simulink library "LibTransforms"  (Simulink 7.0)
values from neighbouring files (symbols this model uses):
  a0 = 0.0    (= 0)    [quake.m]    (also in rampth.m = omega^3; rspect.m = 1; displA2T.m = positT2A(zeros(ntbl, 1), dof, rh, rb, rl, canon, atype); displEnvelope.m = varargin{1}{7})
  atype = []    [displA2T.m]    (also in displEnvelope.m = varargin{1}{6}; displJacobian.m = ones(nact, 1); displT2A.m; forceA2T.m)
  canon = [linDisplCanon linVelocCanon linAccelCanon linForceCanon  		 rotDisplCanon rotVelocCanon rotAccelCanon rotForceCanon]'    [initialize.m]    (also in accelEnvelope.m = varargin{1}{4}; displEnvelope.m = varargin{1}{5}; displPivotEnvelope.m = varargin{1}{6}; forceEnvelope.m = varargin{1}{6})
  dmax = ( (stroke2 + endLength2) * lengthCanon)'    [initialize.m]
  dof = [1 2]    [initialize.m]    (also in accelEnvelope.m = varargin{1}{1}; displEnvelope.m = varargin{1}{1}; displPivotEnvelope.m = varargin{1}{1}; forceEnvelope.m = varargin{1}{2})
  ea = dcm * ea    [initialize.m]    (also in accelEnvelope.m = varargin{1}{3})
  fmax = ( area1 * areaCanon * (supplyPress-returnPress) * pressCanon)'    [initialize.m]    (also in Tutorial.m = 50; forceEnvelope.m = varargin{1}{10}; forceJacobian.m = []; forceT2A.m = [])
  gee = geeCanon / linAccelCanon * 0    (= 0)    [initialize.m]    (also in accelA2T.m; accelEnvelope.m = varargin{1}{6}; accelT2A.m)
  linAccelCanon = 9810.0    (= 9810)    [initialize.m]    (also in accelJacobian.m = canon(3); accelP2Q.m = canon(3))
  linDisplCanon = 1    [initialize.m]    (also in displJacobian.m = canon(1); velocJacobian.m = canon(1))
  linVelocCanon = 1000.0    (= 1000)    [initialize.m]    (also in forceInvJacobian.m = canon(2); velocJacobian.m = canon(2); velocP2Q.m = canon(2))
  ra = dcm * ra    [initialize.m]    (also in accelEnvelope.m = varargin{1}{2})
  rb = dcm * rb    [initialize.m]    (also in displEnvelope.m = varargin{1}{3}; displPivotEnvelope.m = varargin{1}{3}; forceEnvelope.m = varargin{1}{4}; velocEnvelope.m = varargin{1}{4})
  rh = dcm * rh    [initialize.m]    (also in displEnvelope.m = varargin{1}{2}; displPivotEnvelope.m = varargin{1}{2}; forceEnvelope.m = varargin{1}{3}; velocEnvelope.m = varargin{1}{3})
  rl = dcm * rl    [initialize.m]    (also in displEnvelope.m = varargin{1}{4}; displPivotEnvelope.m = varargin{1}{4}; forceEnvelope.m = varargin{1}{5}; velocEnvelope.m = varargin{1}{5})
  rotAccelCanon = pi/180    (= 0.0174532925199)    [initialize.m]    (also in accelJacobian.m = canon(7); accelP2Q.m = canon(7); bodyAccel.m = canon(3); eulerAccel.m = canon(3))
  rotDisplCanon = pi/180    (= 0.0174532925199)    [initialize.m]    (also in accelA2T.m = canon(5); accelP2Q.m = canon(5); accelT2A.m = canon(5); bodyAccel.m = canon(1))
  rotForceCanon = 1000    [initialize.m]    (also in forceInvJacobian.m = canon(8); forceP2Q.m = canon(8))
  rotVelocCanon = pi/180    (= 0.0174532925199)    [initialize.m]    (also in accelJacobian.m = canon(6); accelP2Q.m = canon(6); bodyAccel.m = canon(2); eulerAccel.m = canon(2))
  rows = size(header, 1)    [player.m]    (also in quake.m; savebin.m; viewer.m; accelA2T.m = size(vrot, 1))
  rpq = rpq(:)    [accelP2Q.m]    (also in displP2Q.m; forceP2Q.m; velocP2Q.m)
undefined symbols (not defined in the file or in its folder): aijac, ajac, cols, Column, D, magnitude, matrix, vector
libraries: LibTransforms x99, aerospace x9, simulink x6
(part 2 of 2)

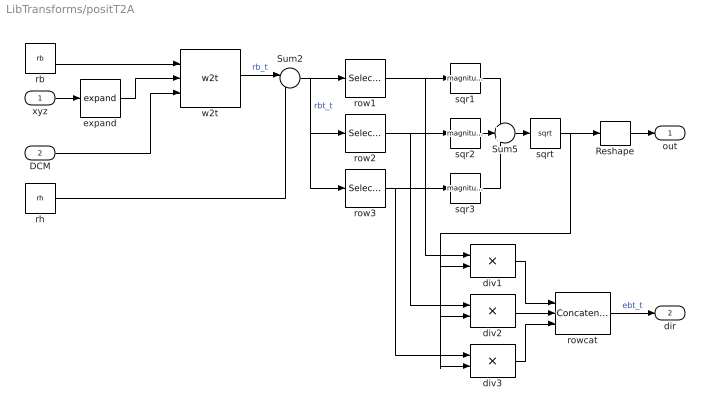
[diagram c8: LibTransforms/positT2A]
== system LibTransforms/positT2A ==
  xyz : Inport  OutDataType=sfix(16)  OutScaling=2^0
  DCM : Inport  Port=2  OutDataType=sfix(16)  OutScaling=2^0
  Reshape : Reshape
  Sum2 : Sum  Inputs=|-+  OutDataType=sfix(16)  OutScaling=2^0
  Sum5 : Sum  Inputs=+++  OutDataType=sfix(16)  OutScaling=2^0
  div1 : Product  Inputs=*/  OutDataType=sfix(16)  OutScaling=2^0
  div2 : Product  Inputs=*/  OutDataType=sfix(16)  OutScaling=2^0
  div3 : Product  Inputs=*/  OutDataType=sfix(16)  OutScaling=2^0
  expand : LibTransforms/expand  SystemSampleTime=-1  size=3  elements=dof(find(dof<=3))
  rb : Constant  Value=rb  OutDataType=sfix(16)  OutScaling=2^0
  rh : Constant  Value=rh  OutDataType=sfix(16)  OutScaling=2^0
  row1 : Selector  NumberOfDimensions=2  InputPortWidth=3  IndexOptions=Index vector (dialog),Select all  Indices=1,-1  OutputSizes=1
  row2 : Selector  NumberOfDimensions=2  InputPortWidth=3  IndexOptions=Index vector (dialog),Select all  Indices=2,-1  OutputSizes=1
  row3 : Selector  NumberOfDimensions=2  InputPortWidth=3  IndexOptions=Index vector (dialog),Select all  Indices=3,-1  OutputSizes=1
  rowcat : Concatenate  NumInputs=3  Mode=Multidimensional array
  sqr1 : Math  Operator=magnitude^2  OutDataType=sfix(16)  OutScaling=2^0
  sqr2 : Math  Operator=magnitude^2  OutDataType=sfix(16)  OutScaling=2^0
  sqr3 : Math  Operator=magnitude^2  OutDataType=sfix(16)  OutScaling=2^0
  sqrt : Math  Operator=sqrt  OutDataType=sfix(16)  OutScaling=2^0
  w2t : LibTransforms/w2t  SystemSampleTime=-1
  out : Outport  OutDataType=sfix(16)  OutScaling=2^0
  dir : Outport  Port=2  OutDataType=sfix(16)  OutScaling=2^0
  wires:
  expand/1 -> w2t/2
  xyz/1 -> expand/1
  rb/1 -> w2t/1
  rh/1 -> Sum2/2
  row2/1 -> sqr2/1, div2/1
  row1/1 -> sqr1/1, div1/1
  row3/1 -> sqr3/1, div3/1
  Sum5/1 -> sqrt/1
  sqrt/1 -> div1/2, div2/2, div3/2, Reshape/1
  w2t/1 -> Sum2/1  "rb_t"
  Sum2/1 -> row3/1, row2/1, row1/1  "rbt_t"
  sqr1/1 -> Sum5/1
  sqr2/1 -> Sum5/2
  sqr3/1 -> Sum5/3
  rowcat/1 -> dir/1  "ebt_t"
  div1/1 -> rowcat/1
  div2/1 -> rowcat/2
  div3/1 -> rowcat/3
  DCM/1 -> w2t/3
  Reshape/1 -> out/1

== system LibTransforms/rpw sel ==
  inp : Inport  OutDataType=sfix(16)  OutScaling=2^0
  Selector : Selector  IndexOptions=Index vector (dialog)  Indices=elements  OutputSizes=1
  out : Outport  OutDataType=sfix(16)  OutScaling=2^0
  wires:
  inp/1 -> Selector/1
  Selector/1 -> out/1

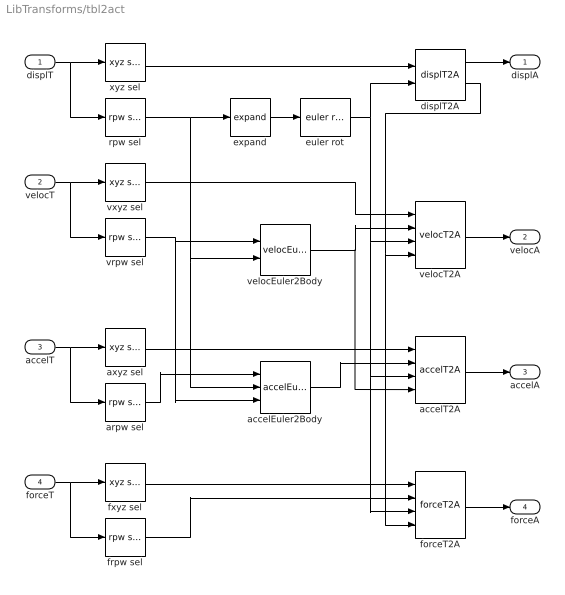
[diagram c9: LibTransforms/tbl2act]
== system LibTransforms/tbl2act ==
  displT : Inport  OutDataType=sfix(16)  OutScaling=2^0
  velocT : Inport  Port=2  OutDataType=sfix(16)  OutScaling=2^0
  accelT : Inport  Port=3  OutDataType=sfix(16)  OutScaling=2^0
  forceT : Inport  Port=4  OutDataType=sfix(16)  OutScaling=2^0
  accelEuler2Body : LibTransforms/accelEuler2Body  SystemSampleTime=-1  dof=dof
  accelT2A : LibTransforms/accelT2A  SystemSampleTime=-1  dof=dof  ra=ra  ea=ea  jac=ajac  gee=gee
  arpw sel : LibTransforms/rpw sel  SystemSampleTime=-1  dof=dof
  axyz sel : LibTransforms/xyz sel  SystemSampleTime=-1  dof=dof
  displT2A : LibTransforms/displT2A  SystemSampleTime=-1  dof=dof  rh=rh  rb=rb  a0=a0
  euler rot : LibTransforms/euler rot  SystemSampleTime=-1
  expand : LibTransforms/expand  SystemSampleTime=-1  size=3  elements=dof(find(dof>3))-3
  forceT2A : LibTransforms/forceT2A  SystemSampleTime=-1  dof=dof  rh=rh
  frpw sel : LibTransforms/rpw sel  SystemSampleTime=-1  dof=dof
  fxyz sel : LibTransforms/xyz sel  SystemSampleTime=-1  dof=dof
  rpw sel : LibTransforms/rpw sel  SystemSampleTime=-1  dof=dof
  velocEuler2Body : LibTransforms/velocEuler2Body  SystemSampleTime=-1  dof=dof
  velocT2A : LibTransforms/velocT2A  SystemSampleTime=-1  dof=dof  rh=rh
  vrpw sel : LibTransforms/rpw sel  SystemSampleTime=-1  dof=dof
  vxyz sel : LibTransforms/xyz sel  SystemSampleTime=-1  dof=dof
  xyz sel : LibTransforms/xyz sel  SystemSampleTime=-1  dof=dof
  displA : Outport  OutDataType=sfix(16)  OutScaling=2^0
  velocA : Outport  Port=2  OutDataType=sfix(16)  OutScaling=2^0
  accelA : Outport  Port=3  OutDataType=sfix(16)  OutScaling=2^0
  forceA : Outport  Port=4  OutDataType=sfix(16)  OutScaling=2^0
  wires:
  expand/1 -> euler rot/1
  xyz sel/1 -> displT2A/1
  displT/1 -> xyz sel/1, rpw sel/1
  rpw sel/1 -> expand/1, velocEuler2Body/2, accelEuler2Body/2
  euler rot/1 -> displT2A/2, accelT2A/3, forceT2A/3, velocT2A/3
  axyz sel/1 -> accelT2A/1
  accelT/1 -> arpw sel/1, axyz sel/1
  displT2A/2 -> forceT2A/4, velocT2A/4
  displT2A/1 -> displA/1
  forceT2A/1 -> forceA/1
  forceT/1 -> frpw sel/1, fxyz sel/1
  fxyz sel/1 -> forceT2A/1
  frpw sel/1 -> forceT2A/2
  velocEuler2Body/1 -> accelT2A/4, velocT2A/2
  accelEuler2Body/1 -> accelT2A/2
  arpw sel/1 -> accelEuler2Body/1
  accelT2A/1 -> accelA/1
  velocT/1 -> vrpw sel/1, vxyz sel/1
  vrpw sel/1 -> velocEuler2Body/1, accelEuler2Body/3
  velocT2A/1 -> velocA/1
  vxyz sel/1 -> velocT2A/1

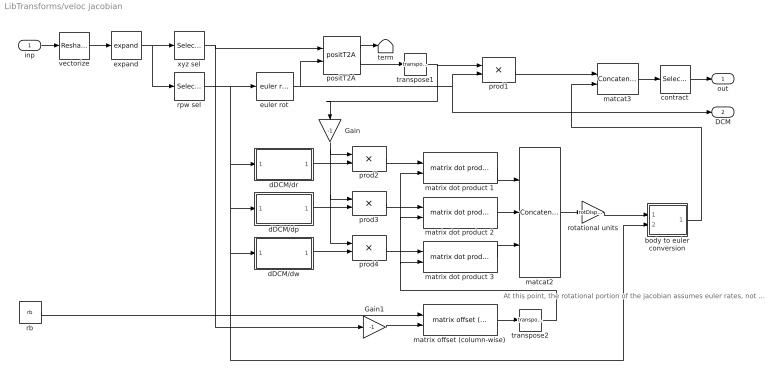
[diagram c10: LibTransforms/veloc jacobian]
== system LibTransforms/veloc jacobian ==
  note: At this point, the rotational portion of the jacobian assumes euler rates, not body rates. To convert it to use body rates, blend the body-to-euler transformation matrix into the rotational portion.
  inp : Inport  OutDataType=sfix(16)  OutScaling=2^0
  Gain : Gain  Orientation=down  Gain=-1  ParameterDataType=sfix(16)  ParameterScaling=2^0  OutDataType=sfix(16)  OutScaling=2^0
  Gain1 : Gain  Gain=-1  ParameterDataType=sfix(16)  ParameterScaling=2^0  OutDataType=sfix(16)  OutScaling=2^0
  body to euler conversion : Subsystem
  contract : Selector  NumberOfDimensions=2  InputPortWidth=3  IndexOptions=Select all,Index vector (dialog)  Indices=-1,dof  OutputSizes=1
  dDCM/dp : Subsystem
  dDCM/dr : Subsystem
  dDCM/dw : Subsystem
  euler rot : LibTransforms/euler rot  SystemSampleTime=-1
  expand : LibTransforms/expand  SystemSampleTime=-1  size=6  elements=dof
  matcat2 : Concatenate  NumInputs=3  Mode=Multidimensional array  ConcatenateDimension=2
  matcat3 : Concatenate  Mode=Multidimensional array  ConcatenateDimension=2
  matrix dot product 1 : LibTransforms/matrix dot product (row-wise)  SystemSampleTime=-1  rows=size(rh,2)
  matrix dot product 2 : LibTransforms/matrix dot product (row-wise)  SystemSampleTime=-1  rows=size(rh,2)
  matrix dot product 3 : LibTransforms/matrix dot product (row-wise)  SystemSampleTime=-1  rows=size(rh,2)
  matrix offset (column-wise) : LibTransforms/matrix offset (column-wise)  SystemSampleTime=-1  cols=size(rh,2)
  positT2A : LibTransforms/positT2A  SystemSampleTime=-1  dof=1:6  rh=rh  rb=rb
  prod{1..4} (4 alike) : Product  Multiplication=Matrix(*)  OutDataType=sfix(16)  OutScaling=2^0
  rb : Constant  Value=rb  OutDataType=sfix(16)  OutScaling=2^0
  rotational units : Gain  Gain=rotDisplCanon * (linDisplCanon/rotDisplCanon) * (rotVelocCanon/linVelocCanon)  ParameterDataType=sfix(16)  ParameterScaling=2^0  OutDataType=sfix(16)  OutScaling=2^0
  rpw sel : Selector  IndexOptions=Index vector (dialog)  Indices=[4 5 6]  OutputSizes=1
  term : Terminator
  transpose1 : Math  Operator=transpose  OutDataType=sfix(16)  OutScaling=2^0
  transpose2 : Math  Operator=transpose  OutDataType=sfix(16)  OutScaling=2^0
  vectorize : Reshape  OutputDimensionality=Column vector (2-D)  OutputDimensions=[3,3]
  xyz sel : Selector  IndexOptions=Index vector (dialog)  Indices=[1 2 3]  OutputSizes=1
  out : Outport  OutDataType=sfix(16)  OutScaling=2^0
  DCM : Outport  Port=2  OutDataType=sfix(16)  OutScaling=2^0
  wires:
  body to euler conversion/1(out) -> matcat3/2
  rb/1 -> matrix offset (column-wise)/1
  Gain1/1 -> matrix offset (column-wise)/2
  transpose2/1 -> matrix dot product 3/2, matrix dot product 2/2, matrix dot product 1/2
  rotational units/1 -> body to euler conversion/1(inp)
  matrix dot product 3/1 -> matcat2/3
  matrix dot product 2/1 -> matcat2/2
  matrix dot product 1/1 -> matcat2/1
  inp/1 -> vectorize/1
  rpw sel/1 -> body to euler conversion/2(rpw), dDCM/dw/1(rpw), dDCM/dp/1(rpw), dDCM/dr/1(rpw), euler rot/1
  euler rot/1 -> positT2A/2, prod1/2, DCM/1
  xyz sel/1 -> positT2A/1, Gain1/1
  positT2A/1 -> term/1
  dDCM/dr/1(dDCM/dr) -> prod2/2
  dDCM/dw/1(dDCM/dw) -> prod4/2
  dDCM/dp/1(dDCM/dp) -> prod3/2
  matrix offset (column-wise)/1 -> transpose2/1
  prod2/1 -> matrix dot product 1/1
  prod3/1 -> matrix dot product 2/1
  prod4/1 -> matrix dot product 3/1
  matcat2/1 -> rotational units/1
  prod1/1 -> matcat3/1
  matcat3/1 -> contract/1
  Gain/1 -> prod4/1, prod3/1, prod2/1
  positT2A/2 -> transpose1/1
  transpose1/1 -> prod1/1, Gain/1
  expand/1 -> rpw sel/1, xyz sel/1
  contract/1 -> out/1
  vectorize/1 -> expand/1

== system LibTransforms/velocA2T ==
  inp : Inport  OutDataType=sfix(16)  OutScaling=2^0
  dinp : Inport  Port=2  OutDataType=sfix(16)  OutScaling=2^0
  Terminator : Terminator
  matrix inverse : LibTransforms/matrix inverse  SystemSampleTime=-1  rows=size(rh, 2)  cols=length(dof)  wate=[]
  prod : Product  Multiplication=Matrix(*)  OutDataType=sfix(16)  OutScaling=2^0
  rpw sel : LibTransforms/rpw sel  SystemSampleTime=-1  dof=dof
  veloc jacobian : LibTransforms/veloc jacobian  SystemSampleTime=-1  dof=dof  rh=rh  rb=rb
  xyz sel : LibTransforms/xyz sel  SystemSampleTime=-1  dof=dof
  xyz : Outport  OutDataType=sfix(16)  OutScaling=2^0
  rpw : Outport  Port=2  OutDataType=sfix(16)  OutScaling=2^0
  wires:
  rpw sel/1 -> rpw/1
  prod/1 -> rpw sel/1, xyz sel/1
  matrix inverse/1 -> prod/1
  veloc jacobian/1 -> matrix inverse/1
  veloc jacobian/2 -> Terminator/1
  xyz sel/1 -> xyz/1
  dinp/1 -> veloc jacobian/1
  inp/1 -> prod/2

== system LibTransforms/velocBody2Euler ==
  inp : Inport  OutDataType=sfix(16)  OutScaling=2^0
  rpw : Inport  Port=2  OutDataType=sfix(16)  OutScaling=2^0
  contract : LibTransforms/contract  SystemSampleTime=-1  elements=[dof(find(dof>3))-3]
  euler rate : LibTransforms/euler rate  SystemSampleTime=-1
  expand 1 : LibTransforms/expand  SystemSampleTime=-1  size=3  elements=dof(find(dof>3))-3
  expand 2 : LibTransforms/expand  SystemSampleTime=-1  size=3  elements=dof(find(dof>3))-3
  out : Outport  OutDataType=sfix(16)  OutScaling=2^0
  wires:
  expand 2/1 -> euler rate/2
  expand 1/1 -> euler rate/1
  contract/1 -> out/1
  rpw/1 -> expand 2/1
  inp/1 -> expand 1/1
  euler rate/1 -> contract/1

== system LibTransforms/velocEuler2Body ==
  inp : Inport  OutDataType=sfix(16)  OutScaling=2^0
  rpw : Inport  Port=2  OutDataType=sfix(16)  OutScaling=2^0
  body rate : LibTransforms/body rate  SystemSampleTime=-1
  contract : LibTransforms/contract  SystemSampleTime=-1  elements=[dof(find(dof>3))-3]
  expand 1 : LibTransforms/expand  SystemSampleTime=-1  size=3  elements=dof(find(dof>3))-3
  expand 2 : LibTransforms/expand  SystemSampleTime=-1  size=3  elements=dof(find(dof>3))-3
  out : Outport  OutDataType=sfix(16)  OutScaling=2^0
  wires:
  body rate/1 -> contract/1
  inp/1 -> expand 1/1
  rpw/1 -> expand 2/1
  contract/1 -> out/1
  expand 1/1 -> body rate/1
  expand 2/1 -> body rate/2

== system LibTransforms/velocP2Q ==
  xyz : Inport  OutDataType=sfix(16)  OutScaling=2^0
  rpw : Inport  Port=2  OutDataType=sfix(16)  OutScaling=2^0
  DCM : Inport  Port=3  OutDataType=sfix(16)  OutScaling=2^0
  Sum : Sum  Inputs=++|  OutDataType=sfix(16)  OutScaling=2^0
  contract : LibTransforms/contract  SystemSampleTime=-1  elements=dof(find(dof<=3))
  crossprod : aerospace/Axes Transformations/3x3 cross product  SystemSampleTime=-1
  expand rpw : LibTransforms/expand  SystemSampleTime=-1  size=3  elements=dof(find(dof>3)) - 3
  expand xyz : LibTransforms/expand  SystemSampleTime=-1  size=3  elements=dof(find(dof<=3))
  linVelocUnits : Gain  Gain=1/linVelocCanon  ParameterDataType=sfix(16)  ParameterScaling=2^0  OutDataType=sfix(16)  OutScaling=2^0
  origin offset : Constant  Value=ofst  OutDataType=sfix(16)  OutScaling=2^0
  prod : Product  Multiplication=Matrix(*)  OutDataType=sfix(16)  OutScaling=2^0
  rotVelocCanon : Gain  Gain=rotVelocCanon  ParameterDataType=sfix(16)  ParameterScaling=2^0  OutDataType=sfix(16)  OutScaling=2^0
  t2w : Math  Operator=transpose  OutDataType=sfix(16)  OutScaling=2^0
  out : Outport  OutDataType=sfix(16)  OutScaling=2^0
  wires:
  xyz/1 -> expand xyz/1
  linVelocUnits/1 -> Sum/2
  origin offset/1 -> crossprod/2
  expand rpw/1 -> crossprod/1
  rotVelocCanon/1 -> expand rpw/1
  rpw/1 -> rotVelocCanon/1
  DCM/1 -> t2w/1
  Sum/1 -> contract/1
  crossprod/1 -> prod/2
  t2w/1 -> prod/1
  expand xyz/1 -> Sum/1
  prod/1 -> linVelocUnits/1
  contract/1 -> out/1

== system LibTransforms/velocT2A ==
  xyz : Inport  OutDataType=sfix(16)  OutScaling=2^0
  rpw : Inport  Port=2  OutDataType=sfix(16)  OutScaling=2^0
  DCM : Inport  Port=3  OutDataType=sfix(16)  OutScaling=2^0
  dir : Inport  Port=4  OutDataType=sfix(16)  OutScaling=2^0
  subsystem : Subsystem
  out : Outport  OutDataType=sfix(16)  OutScaling=2^0
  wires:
  subsystem/1(out) -> out/1
  dir/1 -> subsystem/4(dir)
  xyz/1 -> subsystem/1(xyz)
  rpw/1 -> subsystem/2(rpw)
  DCM/1 -> subsystem/3(DCM)

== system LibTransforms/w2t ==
  inp : Inport  OutDataType=sfix(16)  OutScaling=2^0
  xyz : Inport  Port=2  OutDataType=sfix(16)  OutScaling=2^0
  DCM : Inport  Port=3  OutDataType=sfix(16)  OutScaling=2^0
  Demux : Demux  Outputs=3
  Sum5 : Sum  Inputs=-+|  OutDataType=sfix(16)  OutScaling=2^0
  Sum6 : Sum  Inputs=-+|  OutDataType=sfix(16)  OutScaling=2^0
  Sum7 : Sum  Inputs=-+|  OutDataType=sfix(16)  OutScaling=2^0
  prod : Product  Multiplication=Matrix(*)  OutDataType=sfix(16)  OutScaling=2^0
  row1A : Selector  NumberOfDimensions=2  InputPortWidth=3  IndexOptions=Index vector (dialog),Select all  Indices=1,-1  OutputSizes=1
  row2A : Selector  NumberOfDimensions=2  InputPortWidth=3  IndexOptions=Index vector (dialog),Select all  Indices=2,-1  OutputSizes=1
  row3A : Selector  NumberOfDimensions=2  InputPortWidth=3  IndexOptions=Index vector (dialog),Select all  Indices=3,-1  OutputSizes=1
  rowcat : Concatenate  NumInputs=3  Mode=Multidimensional array
  out : Outport  OutDataType=sfix(16)  OutScaling=2^0
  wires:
  Sum7/1 -> rowcat/3
  Sum5/1 -> rowcat/1
  Sum6/1 -> rowcat/2
  Demux/3 -> Sum7/1
  Demux/2 -> Sum6/1
  row3A/1 -> Sum7/2
  row2A/1 -> Sum6/2
  Demux/1 -> Sum5/1
  row1A/1 -> Sum5/2
  xyz/1 -> Demux/1
  inp/1 -> row1A/1, row2A/1, row3A/1
  rowcat/1 -> prod/2
  prod/1 -> out/1
  DCM/1 -> prod/1

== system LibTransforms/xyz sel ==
  inp : Inport  OutDataType=sfix(16)  OutScaling=2^0
  Selector : Selector  IndexOptions=Index vector (dialog)  Indices=elements  OutputSizes=1
  out : Outport  OutDataType=sfix(16)  OutScaling=2^0
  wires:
  Selector/1 -> out/1
  inp/1 -> Selector/1

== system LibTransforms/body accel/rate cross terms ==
  inp : Inport  OutDataType=sfix(16)  OutScaling=2^0
  13 : Fcn  Expr=-cos(u[2])*u[5]*u[6]
  23 : Fcn  Expr=-sin(u[1])*u[4]*u[5] + cos(u[1])*cos(u[2])*u[4]*u[6] - sin(u[1])*sin(u[2])*u[5]*u[6]
  33 : Fcn  Expr=-cos(u[1])*u[4]*u[5] - sin(u[1])*cos(u[2])*u[4]*u[6] - cos(u[1])*sin(u[2])*u[5]*u[6]
  Mux : Mux  Inputs=3
  out : Outport  OutDataType=sfix(16)  OutScaling=2^0
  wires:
  Mux/1 -> out/1
  33/1 -> Mux/3
  23/1 -> Mux/2
  13/1 -> Mux/1
  inp/1 -> 33/1, 23/1, 13/1

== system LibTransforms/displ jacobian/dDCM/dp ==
  rpw : Inport  OutDataType=sfix(16)  OutScaling=2^0
  11 : Fcn  Expr=-sin(u[2])*cos(u[3])
  12 : Fcn  Expr=-sin(u[2])*sin(u[3])
  13 : Fcn  Expr=-cos(u[2])
  21 : Fcn  Expr=sin(u[1])*cos(u[2])*cos(u[3])
  22 : Fcn  Expr=sin(u[1])*cos(u[2])*sin(u[3])
  23 : Fcn  Expr=-sin(u[1])*sin(u[2])
  31 : Fcn  Expr=cos(u[1])*cos(u[2])*cos(u[3])
  32 : Fcn  Expr=cos(u[1])*cos(u[2])*sin(u[3])
  33 : Fcn  Expr=-cos(u[1])*sin(u[2])
  9x1->3x3 : simulink/Math Operations/Reshape  OutputDimensionality=Customize  OutputDimensions=[3,3]
  Mux2 : Mux  Orientation=down  Inputs=9
  rotDisplCanon : Gain  Gain=rotDisplCanon  ParameterDataType=sfix(16)  ParameterScaling=2^0  OutDataType=sfix(16)  OutScaling=2^0
  dDCM/dp : Outport  OutDataType=sfix(16)  OutScaling=2^0
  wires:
  rotDisplCanon/1 -> 31/1, 21/1, 11/1, 32/1, 22/1, 12/1, 33/1, 23/1, 13/1
  9x1->3x3/1 -> dDCM/dp/1
  11/1 -> Mux2/1
  21/1 -> Mux2/2
  31/1 -> Mux2/3
  rpw/1 -> rotDisplCanon/1
  12/1 -> Mux2/4
  22/1 -> Mux2/5
  32/1 -> Mux2/6
  Mux2/1 -> 9x1->3x3/1
  13/1 -> Mux2/7
  23/1 -> Mux2/8
  33/1 -> Mux2/9

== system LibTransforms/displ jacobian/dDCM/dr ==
  rpw : Inport  OutDataType=sfix(16)  OutScaling=2^0
  11 : Fcn  Expr=0
  12 : Fcn  Expr=0
  13 : Fcn  Expr=0
  21 : Fcn  Expr=cos(u[1])*sin(u[2])*cos(u[3])+sin(u[1])*sin(u[3])
  22 : Fcn  Expr=cos(u[1])*sin(u[2])*sin(u[3])-sin(u[1])*cos(u[3])
  23 : Fcn  Expr=cos(u[1])*cos(u[2])
  31 : Fcn  Expr=-sin(u[1])*sin(u[2])*cos(u[3])+cos(u[1])*sin(u[3])
  32 : Fcn  Expr=-sin(u[1])*sin(u[2])*sin(u[3])-cos(u[1])*cos(u[3])
  33 : Fcn  Expr=-sin(u[1])*cos(u[2])
  9x1->3x3 : simulink/Math Operations/Reshape  OutputDimensionality=Customize  OutputDimensions=[3,3]
  Mux2 : Mux  Orientation=down  Inputs=9
  rotDisplCanon : Gain  Gain=rotDisplCanon  ParameterDataType=sfix(16)  ParameterScaling=2^0  OutDataType=sfix(16)  OutScaling=2^0
  dDCM/dr : Outport  OutDataType=sfix(16)  OutScaling=2^0
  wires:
  rotDisplCanon/1 -> 31/1, 21/1, 11/1, 32/1, 22/1, 12/1, 33/1, 23/1, 13/1
  9x1->3x3/1 -> dDCM/dr/1
  11/1 -> Mux2/1
  21/1 -> Mux2/2
  31/1 -> Mux2/3
  rpw/1 -> rotDisplCanon/1
  12/1 -> Mux2/4
  22/1 -> Mux2/5
  32/1 -> Mux2/6
  Mux2/1 -> 9x1->3x3/1
  13/1 -> Mux2/7
  23/1 -> Mux2/8
  33/1 -> Mux2/9

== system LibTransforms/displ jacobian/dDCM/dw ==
  rpw : Inport  OutDataType=sfix(16)  OutScaling=2^0
  11 : Fcn  Expr=-cos(u[2])*sin(u[3])
  12 : Fcn  Expr=cos(u[2])*cos(u[3])
  13 : Fcn  Expr=0
  21 : Fcn  Expr=-sin(u[1])*sin(u[2])*sin(u[3])-cos(u[1])*cos(u[3])
  22 : Fcn  Expr=sin(u[1])*sin(u[2])*cos(u[3])-cos(u[1])*sin(u[3])
  23 : Fcn  Expr=0
  31 : Fcn  Expr=-cos(u[1])*sin(u[2])*sin(u[3])+sin(u[1])*cos(u[3])
  32 : Fcn  Expr=cos(u[1])*sin(u[2])*cos(u[3])+sin(u[1])*sin(u[3])
  33 : Fcn  Expr=0
  9x1->3x3 : simulink/Math Operations/Reshape  OutputDimensionality=Customize  OutputDimensions=[3,3]
  Mux2 : Mux  Orientation=down  Inputs=9
  rotDisplCanon : Gain  Gain=rotDisplCanon  ParameterDataType=sfix(16)  ParameterScaling=2^0  OutDataType=sfix(16)  OutScaling=2^0
  dDCM/dw : Outport  OutDataType=sfix(16)  OutScaling=2^0
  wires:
  rotDisplCanon/1 -> 31/1, 21/1, 11/1, 32/1, 22/1, 12/1, 33/1, 23/1, 13/1
  9x1->3x3/1 -> dDCM/dw/1
  11/1 -> Mux2/1
  21/1 -> Mux2/2
  31/1 -> Mux2/3
  rpw/1 -> rotDisplCanon/1
  12/1 -> Mux2/4
  22/1 -> Mux2/5
  32/1 -> Mux2/6
  Mux2/1 -> 9x1->3x3/1
  13/1 -> Mux2/7
  23/1 -> Mux2/8
  33/1 -> Mux2/9

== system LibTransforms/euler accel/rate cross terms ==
  inp : Inport  OutDataType=sfix(16)  OutScaling=2^0
  13 : Fcn  Expr=tan(u[2])*u[4]*u[5] + (1/cos(u[2]))*u[5]*u[6]
  23 : Fcn  Expr=-cos(u[2])*u[4]*u[6]
  33 : Fcn  Expr=tan(u[2])*u[5]*u[6] + (1/cos(u[2]))*u[4]*u[5]
  Mux : Mux  Inputs=3
  out : Outport  OutDataType=sfix(16)  OutScaling=2^0
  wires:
  inp/1 -> 13/1, 23/1, 33/1
  13/1 -> Mux/1
  23/1 -> Mux/2
  33/1 -> Mux/3
  Mux/1 -> out/1

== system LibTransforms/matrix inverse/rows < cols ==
  inp : Inport  OutDataType=sfix(16)  OutScaling=2^0
  Action Port : ActionPort
  Product : Product  Multiplication=Matrix(*)  OutDataType=sfix(16)  OutScaling=2^0
  Product1 : Product  Multiplication=Matrix(*)  OutDataType=sfix(16)  OutScaling=2^0
  Product2 : Product  Multiplication=Matrix(*)  OutDataType=sfix(16)  OutScaling=2^0
  matrix inverse : Product  Inputs=/  Multiplication=Matrix(*)  OutDataType=sfix(16)  OutScaling=2^-10
  transpose1 : Math  Operator=transpose  OutDataType=sfix(16)  OutScaling=2^0
  weight : Constant  Value=w1  OutDataType=sfix(16)  OutScaling=2^0
  out : Outport  OutDataType=sfix(16)  OutScaling=2^0
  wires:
  matrix inverse/1 -> Product1/2
  Product2/1 -> Product1/1, Product/2
  weight/1 -> Product2/1
  transpose1/1 -> Product2/2
  Product/1 -> matrix inverse/1
  inp/1 -> Product/1, transpose1/1
  Product1/1 -> out/1

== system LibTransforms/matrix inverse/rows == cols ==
  inp : Inport  OutDataType=sfix(16)  OutScaling=2^0
  Action Port : ActionPort
  Product : Product  Multiplication=Matrix(*)  OutDataType=sfix(16)  OutScaling=2^0
  Product1 : Product  Multiplication=Matrix(*)  OutDataType=sfix(16)  OutScaling=2^0
  matrix inverse : Product  Inputs=/  Multiplication=Matrix(*)  OutDataType=sfix(16)  OutScaling=2^-10
  transpose1 : Math  Operator=transpose  OutDataType=sfix(16)  OutScaling=2^0
  out : Outport  OutDataType=sfix(16)  OutScaling=2^0
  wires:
  Product/1 -> matrix inverse/1
  inp/1 -> Product/2, transpose1/1
  matrix inverse/1 -> Product1/1
  transpose1/1 -> Product1/2, Product/1
  Product1/1 -> out/1

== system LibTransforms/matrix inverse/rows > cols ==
  inp : Inport  OutDataType=sfix(16)  OutScaling=2^0
  Action Port : ActionPort
  Product : Product  Multiplication=Matrix(*)  OutDataType=sfix(16)  OutScaling=2^0
  Product1 : Product  Multiplication=Matrix(*)  OutDataType=sfix(16)  OutScaling=2^0
  Product2 : Product  Multiplication=Matrix(*)  OutDataType=sfix(16)  OutScaling=2^0
  matrix inverse : Product  Inputs=/  Multiplication=Matrix(*)  OutDataType=sfix(16)  OutScaling=2^-10
  transpose1 : Math  Operator=transpose  OutDataType=sfix(16)  OutScaling=2^0
  weight : Constant  Value=w2  OutDataType=sfix(16)  OutScaling=2^0
  out : Outport  OutDataType=sfix(16)  OutScaling=2^0
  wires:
  matrix inverse/1 -> Product1/1
  Product2/1 -> Product1/2, Product/1
  weight/1 -> Product2/2
  transpose1/1 -> Product2/1
  inp/1 -> Product/2, transpose1/1
  Product/1 -> matrix inverse/1
  Product1/1 -> out/1

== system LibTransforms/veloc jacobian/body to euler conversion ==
  inp : Inport
  rpw : Inport  Port=2
  body2euler : LibTransforms/body2euler  SystemSampleTime=-1
  prod : Product  Multiplication=Matrix(*)  OutDataType=sfix(16)  OutScaling=2^0
  rotDisplCanon : Gain  Gain=rotDisplCanon  ParameterDataType=sfix(16)  ParameterScaling=2^0  OutDataType=sfix(16)  OutScaling=2^0
  out : Outport
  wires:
  rpw/1 -> rotDisplCanon/1
  prod/1 -> out/1
  inp/1 -> prod/1
  body2euler/1 -> prod/2
  rotDisplCanon/1 -> body2euler/1

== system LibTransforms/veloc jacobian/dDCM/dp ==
  rpw : Inport  OutDataType=sfix(16)  OutScaling=2^0
  11 : Fcn  Expr=-sin(u[2])*cos(u[3])
  12 : Fcn  Expr=-sin(u[2])*sin(u[3])
  13 : Fcn  Expr=-cos(u[2])
  21 : Fcn  Expr=sin(u[1])*cos(u[2])*cos(u[3])
  22 : Fcn  Expr=sin(u[1])*cos(u[2])*sin(u[3])
  23 : Fcn  Expr=-sin(u[1])*sin(u[2])
  31 : Fcn  Expr=cos(u[1])*cos(u[2])*cos(u[3])
  32 : Fcn  Expr=cos(u[1])*cos(u[2])*sin(u[3])
  33 : Fcn  Expr=-cos(u[1])*sin(u[2])
  9x1->3x3 : Reshape  OutputDimensionality=Customize  OutputDimensions=[3,3]
  Mux2 : Mux  Orientation=down  Inputs=9
  rotDisplCanon : Gain  Gain=rotDisplCanon  ParameterDataType=sfix(16)  ParameterScaling=2^0  OutDataType=sfix(16)  OutScaling=2^0
  dDCM/dp : Outport  OutDataType=sfix(16)  OutScaling=2^0
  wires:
  33/1 -> Mux2/9
  23/1 -> Mux2/8
  13/1 -> Mux2/7
  Mux2/1 -> 9x1->3x3/1
  32/1 -> Mux2/6
  22/1 -> Mux2/5
  12/1 -> Mux2/4
  rpw/1 -> rotDisplCanon/1
  31/1 -> Mux2/3
  21/1 -> Mux2/2
  11/1 -> Mux2/1
  9x1->3x3/1 -> dDCM/dp/1
  rotDisplCanon/1 -> 13/1, 23/1, 33/1, 12/1, 22/1, 32/1, 11/1, 21/1, 31/1

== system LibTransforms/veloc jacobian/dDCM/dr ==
  rpw : Inport  OutDataType=sfix(16)  OutScaling=2^0
  11 : Fcn  Expr=0
  12 : Fcn  Expr=0
  13 : Fcn  Expr=0
  21 : Fcn  Expr=cos(u[1])*sin(u[2])*cos(u[3])+sin(u[1])*sin(u[3])
  22 : Fcn  Expr=cos(u[1])*sin(u[2])*sin(u[3])-sin(u[1])*cos(u[3])
  23 : Fcn  Expr=cos(u[1])*cos(u[2])
  31 : Fcn  Expr=-sin(u[1])*sin(u[2])*cos(u[3])+cos(u[1])*sin(u[3])
  32 : Fcn  Expr=-sin(u[1])*sin(u[2])*sin(u[3])-cos(u[1])*cos(u[3])
  33 : Fcn  Expr=-sin(u[1])*cos(u[2])
  9x1->3x3 : Reshape  OutputDimensionality=Customize  OutputDimensions=[3,3]
  Mux2 : Mux  Orientation=down  Inputs=9
  rotDisplCanon : Gain  Gain=rotDisplCanon  ParameterDataType=sfix(16)  ParameterScaling=2^0  OutDataType=sfix(16)  OutScaling=2^0
  dDCM/dr : Outport  OutDataType=sfix(16)  OutScaling=2^0
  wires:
  33/1 -> Mux2/9
  23/1 -> Mux2/8
  13/1 -> Mux2/7
  Mux2/1 -> 9x1->3x3/1
  32/1 -> Mux2/6
  22/1 -> Mux2/5
  12/1 -> Mux2/4
  rpw/1 -> rotDisplCanon/1
  31/1 -> Mux2/3
  21/1 -> Mux2/2
  11/1 -> Mux2/1
  9x1->3x3/1 -> dDCM/dr/1
  rotDisplCanon/1 -> 13/1, 23/1, 33/1, 12/1, 22/1, 32/1, 11/1, 21/1, 31/1

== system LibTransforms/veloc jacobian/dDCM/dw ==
  rpw : Inport  OutDataType=sfix(16)  OutScaling=2^0
  11 : Fcn  Expr=-cos(u[2])*sin(u[3])
  12 : Fcn  Expr=cos(u[2])*cos(u[3])
  13 : Fcn  Expr=0
  21 : Fcn  Expr=-sin(u[1])*sin(u[2])*sin(u[3])-cos(u[1])*cos(u[3])
  22 : Fcn  Expr=sin(u[1])*sin(u[2])*cos(u[3])-cos(u[1])*sin(u[3])
  23 : Fcn  Expr=0
  31 : Fcn  Expr=-cos(u[1])*sin(u[2])*sin(u[3])+sin(u[1])*cos(u[3])
  32 : Fcn  Expr=cos(u[1])*sin(u[2])*cos(u[3])+sin(u[1])*sin(u[3])
  33 : Fcn  Expr=0
  9x1->3x3 : Reshape  OutputDimensionality=Customize  OutputDimensions=[3,3]
  Mux2 : Mux  Orientation=down  Inputs=9
  rotDisplCanon : Gain  Gain=rotDisplCanon  ParameterDataType=sfix(16)  ParameterScaling=2^0  OutDataType=sfix(16)  OutScaling=2^0
  dDCM/dw : Outport  OutDataType=sfix(16)  OutScaling=2^0
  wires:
  33/1 -> Mux2/9
  23/1 -> Mux2/8
  13/1 -> Mux2/7
  Mux2/1 -> 9x1->3x3/1
  32/1 -> Mux2/6
  22/1 -> Mux2/5
  12/1 -> Mux2/4
  rpw/1 -> rotDisplCanon/1
  31/1 -> Mux2/3
  21/1 -> Mux2/2
  11/1 -> Mux2/1
  9x1->3x3/1 -> dDCM/dw/1
  rotDisplCanon/1 -> 13/1, 23/1, 33/1, 12/1, 22/1, 32/1, 11/1, 21/1, 31/1

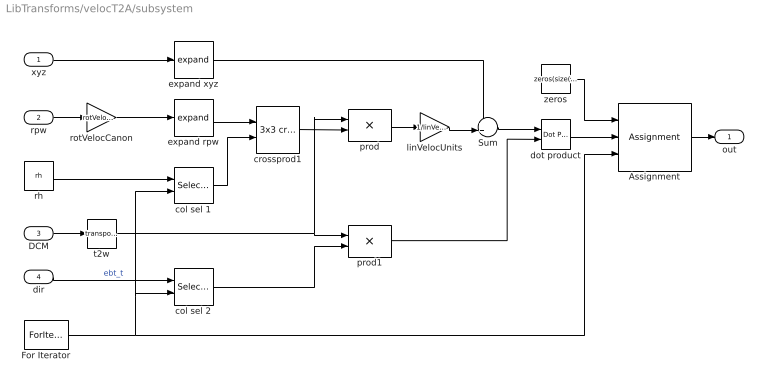
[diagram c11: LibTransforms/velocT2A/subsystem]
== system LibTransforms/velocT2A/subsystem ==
  xyz : Inport  OutDataType=sfix(16)  OutScaling=2^0
  rpw : Inport  Port=2  OutDataType=sfix(16)  OutScaling=2^0
  DCM : Inport  Port=3  OutDataType=sfix(16)  OutScaling=2^0
  dir : Inport  Port=4  OutDataType=sfix(16)  OutScaling=2^0
  Assignment : Assignment  IndexOptions=Index vector (port)  Indices=1  OutputSizes=[1 1]
  For Iterator : ForIterator  IterationLimit=size(rh, 2)
  Sum : Sum  Inputs=++|  OutDataType=sfix(16)  OutScaling=2^0
  col sel 1 : Selector  NumberOfDimensions=2  InputPortWidth=3  IndexOptions=Select all,Index vector (port)  Indices=-1,-1  OutputSizes=1
  col sel 2 : Selector  NumberOfDimensions=2  InputPortWidth=3  IndexOptions=Select all,Index vector (port)  Indices=-1,-1  OutputSizes=1
  crossprod1 : aerospace/Axes Transformations/3x3 cross product  SystemSampleTime=-1
  dot product : simulink/Math Operations/Dot Product  InputSameDT=on  OutDataType=sfix(16)  OutScaling=2^-10  DoSatur=off
  expand rpw : LibTransforms/expand  SystemSampleTime=-1  size=3  elements=dof(find(dof>3)) - 3
  expand xyz : LibTransforms/expand  SystemSampleTime=-1  size=3  elements=dof(find(dof<=3))
  linVelocUnits : Gain  Gain=1/linVelocCanon  ParameterDataType=sfix(16)  ParameterScaling=2^0  OutDataType=sfix(16)  OutScaling=2^0
  prod : Product  Multiplication=Matrix(*)  OutDataType=sfix(16)  OutScaling=2^0
  prod1 : Product  Multiplication=Matrix(*)  OutDataType=sfix(16)  OutScaling=2^0
  rh : Constant  Value=rh  OutDataType=sfix(16)  OutScaling=2^0
  rotVelocCanon : Gain  Gain=rotVelocCanon  ParameterDataType=sfix(16)  ParameterScaling=2^0  OutDataType=sfix(16)  OutScaling=2^0
  t2w : Math  Operator=transpose  OutDataType=sfix(16)  OutScaling=2^0
  zeros : Constant  Value=zeros(size(rh, 2), 1)  OutDataType=sfix(16)  OutScaling=2^0
  out : Outport  OutDataType=sfix(16)  OutScaling=2^0
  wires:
  dir/1 -> col sel 2/1  "ebt_t"
  DCM/1 -> t2w/1
  Assignment/1 -> out/1
  rpw/1 -> rotVelocCanon/1
  xyz/1 -> expand xyz/1
  expand xyz/1 -> Sum/1
  prod1/1 -> dot product/2
  dot product/1 -> Assignment/2
  Sum/1 -> dot product/1
  linVelocUnits/1 -> Sum/2
  col sel 2/1 -> prod1/2
  prod/1 -> linVelocUnits/1
  crossprod1/1 -> prod/2
  For Iterator/1 -> col sel 2/2, col sel 1/2, Assignment/3
  col sel 1/1 -> crossprod1/2
  expand rpw/1 -> crossprod1/1
  rh/1 -> col sel 1/1
  zeros/1 -> Assignment/1
  rotVelocCanon/1 -> expand rpw/1
  t2w/1 -> prod1/1, prod/1
